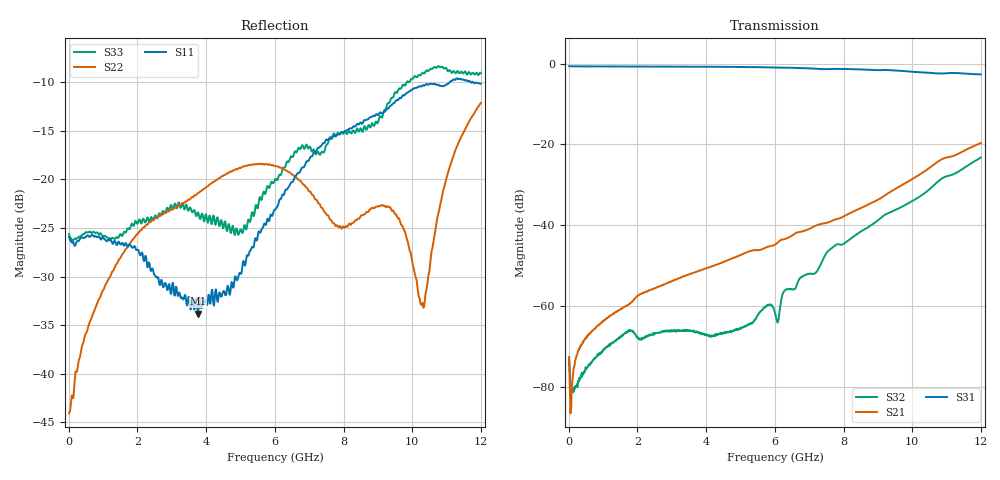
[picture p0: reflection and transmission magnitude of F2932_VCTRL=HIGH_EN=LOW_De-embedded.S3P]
! Integrated Device Technology
! Corporate Headquarters
! 6024 Silver Creek Valley Road
! San Jose, CA 95138  USA
! Phone:  1-408-284-8200
! Toll Free:  1-800-223-1366
! Webpage:  http://www.idt.com/
! Timing and RF Division
! 515 Groton Road, Suite 102
! Westford, MA 01886-6024
! Device:  F2932
! Description: High Reliability SP2T RF Switch
! Frequency:  0.05 -  8.00 GHz
! Package:  4x4 mm QFN Plastic Package: 16 pin
! Ports:  3 RF, 3 DC
!  Pin  1  = VDD
!  Pin  2  = VCTL
!  Pin  3  = RFC  =  Port 3
!  Pin  4  = GND
!  Pin  5  = EN
!  Pin  6  = GND
!  Pin  7  = GND
!  Pin  8  = GND
!  Pin  9  = RF1  =  Port 1
!  Pin 10  = GND
!  Pin 11  = GND
!  Pin  9  = RF2  =  Port 2
!  Pin 13  = GND
!  Pin 14  = GND
!  Pin 15  = GND
!  Pin 16  = NC
! State:  RF1 Selected
! VCTRL:  +2.60 Volts (Logic High)
! EN:  +0.00 Volts (Logic Low)
! Voltage:  +5.00 Volts
! Current:  0.410 mA
! Data:  The device was measured on a F2932 evaluation board which has
!  individual transmission lines to the RF pins.  Data was collected
!  using a calibrated network analyzer.  The evaluation board was
!  de-embedded using AFR (Keysight) technique.
!  The reference plane is the edge of the package pin.
! Misc:
!  Action Tracker AT0443
! Date Measured:  2018-10-10
! Date:  2018-10-11  MJV
! Note:
!  Integrated Device Technology supplies this data as a sample of measured
!  data at the package pin for this product.  Your particular data for this
!  product may vary.
!  Data was taken at 25 degrees C.
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# Hz S dB R 50
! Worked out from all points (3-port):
!   1200 points, 10 MHz to 12 GHz, reference 50 ohm
!   strongest paths, dB at 10 MHz, 3.01 GHz, 6.01 GHz, 9.01 GHz, 12 GHz:
!     S31: -0.6, -0.8, -1.0, -1.6, -2.7
!     S21: -72.5, -53.7, -44.8, -33.6, -19.6
!     S32: -72.9, -66.0, -61.9, -38.7, -23.2
!   lowest |S11| = -33.8 dB at 3.76 GHz (marker M1), VSWR 1.04, Z = 50.4 - j2.02 ohm
!   |S11| at or under -10 dB: start of sweep to 11.09 GHz; 11.70111 GHz to 11.74209 GHz (40.98 MHz wide, 0.35 % of centre); 11.78 GHz to end of sweep
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1e7  -25.91 -3.8  -72.39 -5.6  -0.65 -0.3
     -72.53 -6.1  -44.06 179.1  -73.09 -15.4
     -0.65 -0.3  -72.85 -12.1  -25.61 -3.7
2e8  -26.69 -6.4  -73.13 62.3  -0.70 -3.7
     -72.99 63.4  -39.76 100.8  -79.46 -154.9
     -0.70 -3.7  -79.96 -154.6  -26.09 -7.8
1.42e9  -26.63 -25.7  -61.27 79.9  -0.72 -25.7
        -61.12 78.7  -28.57 50.1  -68.17 98.9
        -0.72 -25.7  -68.08 98.6  -26.00 -32.6
3.76e9  -33.81 -79.0  -51.35 89.3  -0.79 -68.3
        -51.33 89.6  -21.41 24.3  -66.59 25.7
        -0.79 -68.2  -66.52 26.4  -23.37 -78.4
6.01e9  -23.09 161.4  -44.74 95.6  -0.96 -110.9
        -44.75 95.7  -18.60 7.9  -61.79 -129.7
        -0.95 -110.6  -61.90 -129.1  -19.97 -171.2
7.58e9  -15.79 90.4  -39.17 90.4  -1.32 -139.7
        -39.19 90.4  -23.90 -23.1  -46.10 -146.8
        -1.35 -139.5  -46.12 -146.5  -15.87 -175.0
9.39e9  -12.37 65.4  -31.61 85.6  -1.65 -175.9
        -31.58 85.8  -23.11 -103.9  -36.70 168.0
        -1.65 -175.5  -36.63 168.0  -11.64 115.7
1.03e10  -10.33 39.2  -26.97 72.3  -2.18 166.0
         -26.97 72.4  -32.69 175.6  -32.40 152.2
         -2.18 166.5  -32.42 152.1  -9.03 102.4
1.103e10  -10.16 26.9  -23.18 48.3  -2.37 153.7
          -23.18 48.7  -19.46 95.5  -27.80 127.9
          -2.37 154.0  -27.79 128.1  -8.82 94.6
1.2e10  -10.13 8.1  -19.64 19.0  -2.67 131.7
        -19.64 19.4  -12.11 80.5  -23.24 98.3
        -2.69 132.2  -23.22 98.3  -9.06 79.2
